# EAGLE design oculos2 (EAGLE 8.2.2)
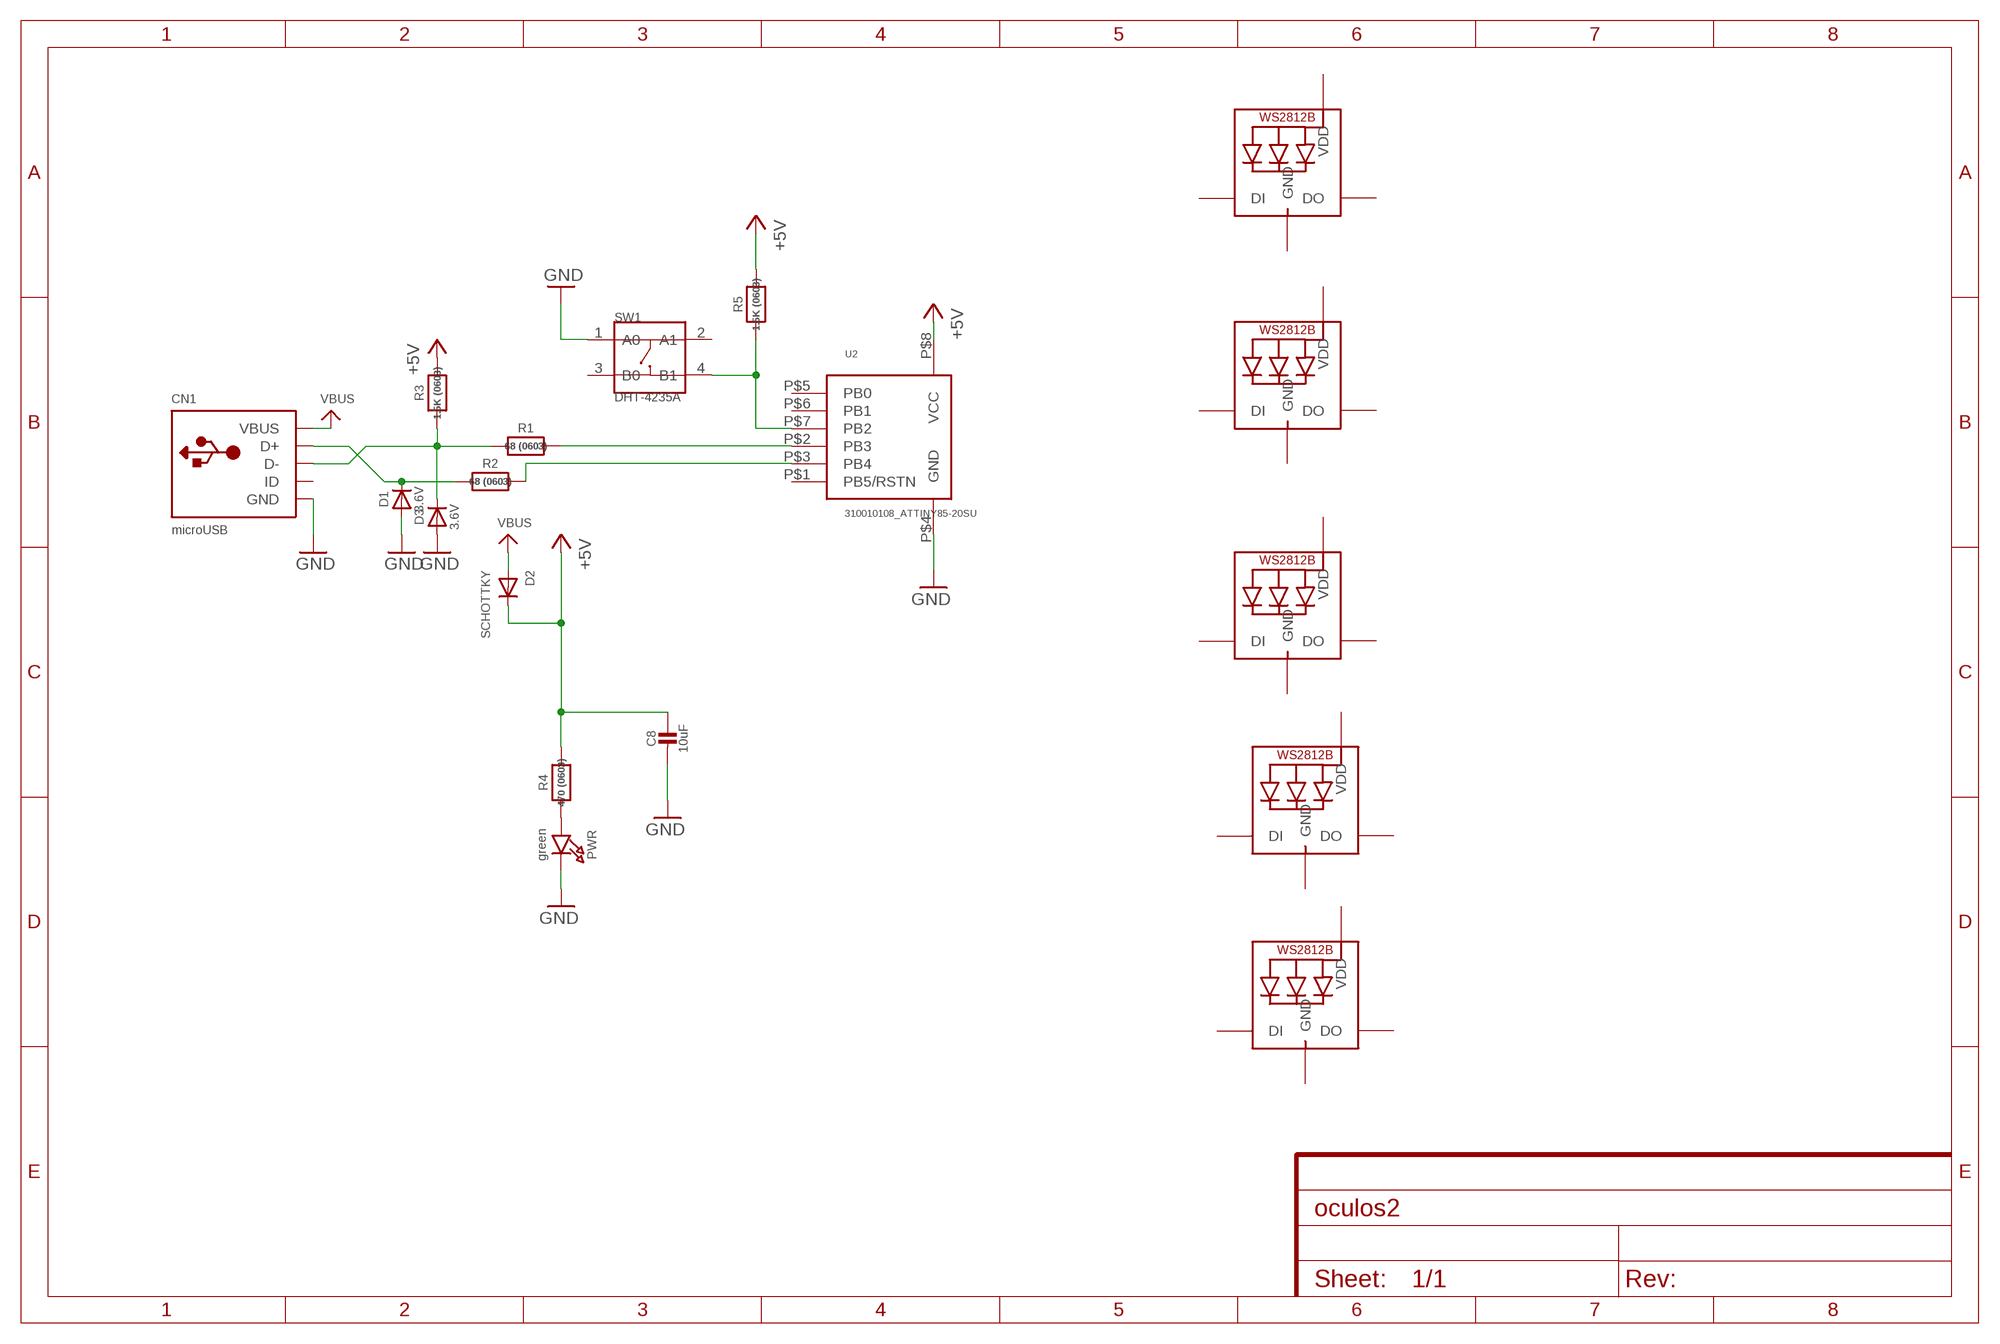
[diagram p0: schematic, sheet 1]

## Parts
C8  10uF  CAP_CERAMIC0805-NOOUTLINE  [0805-NO]
CN1  microUSB  USBMICRO_20329  [4UCONN_20329]
D1  3.6V  DIODESOD-323  [SOD-323]
D2  SCHOTTKY  DIODE_SOD-123FL  [SOD-123FL]
D3  3.6V  DIODESOD-323  [SOD-323]
LED1  WS2812B5050  [WS2812B]
LED2  WS2812B5050  [WS2812B]
LED3  WS2812B5050  [WS2812B]
LED4  WS2812B5050  [WS2812B]
LED5  WS2812B5050  [WS2812B]
PWR  green  LED0805_NOOUTLINE  [CHIPLED_0805_NOOUTLINE]
R1  68 (0603)  RESISTOR_0603_NOOUT  [0603-NO]
R2  68 (0603)  RESISTOR_0603_NOOUT  [0603-NO]
R3  1.5K (0603)  RESISTOR_0603_NOOUT  [0603-NO]
R4  470 (0603)  RESISTOR_0603_NOOUT  [0603-NO]
R5  1.5K (0603)  RESISTOR_0603_NOOUT  [0603-NO]
SW1  DHT-4235A  SMD-BUTTON-TOP-DHT-4235A(4P-4.2X3.2MM)  [SW4-SMD-4.2X3.2X2.5MM]
U2  310010108_ATTINY85-20SU  [SOIC8]

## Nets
+5V: C8.1 D2.C R3.2 R4.2 R5.2 U2.P$8(VCC)
B3: R1.2 U2.P$2(PB3)
GND: C8.2 CN1.BASE@1(GND) CN1.BASE@2(GND) CN1.GND CN1.SPRT@1(GND) CN1.SPRT@2(GND) CN1.SPRT@3(GND) CN1.SPRT@4(GND) D1.A D3.A PWR.C SW1.1(A0) U2.P$4(GND)
N$1: R5.1 SW1.4(B1) U2.P$7(PB2)
N$2: CN1.D+ D1.C R2.1
N$3: R2.2 U2.P$3(PB4)
N$5: CN1.D- D3.C R1.1 R3.1
N$6: PWR.A R4.1
VBUS: CN1.VBUS D2.A
Unconnected: CN1.ID LED1.2-DOUT(DO) LED1.4-DIN(DI) LED2.2-DOUT(DO) LED2.4-DIN(DI) LED3.2-DOUT(DO) LED3.4-DIN(DI) LED4.2-DOUT(DO) LED4.4-DIN(DI) LED5.2-DOUT(DO) LED5.4-DIN(DI) SW1.2(A1) SW1.3(B0) U2.P$1(PB5/RSTN) U2.P$5(PB0) U2.P$6(PB1)

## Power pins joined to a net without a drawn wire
GND: LED1.3-GND(GND) LED2.3-GND(GND) LED3.3-GND(GND) LED4.3-GND(GND) LED5.3-GND(GND)
VDD: LED1.1-VDD(VDD) LED2.1-VDD(VDD) LED3.1-VDD(VDD) LED4.1-VDD(VDD) LED5.1-VDD(VDD)

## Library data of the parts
C8 = microbuilder:CAP_CERAMIC: Ceramic Capacitors
CN1 = microbuilder:USB: USB Connectors USBMINIB - Surface Mount Female Mini-B USB Connector 4UConnector: 06564
D1 D3 = microbuilder:DIODE: Diode
D2 = adafruit:DIODE: Diode
LED1-LED5 = adafruit:WS2812B
PWR = microbuilder:LED: LED
R1-R5 = microbuilder:RESISTOR: Resistors
SW1 = Seeed-Switch-2016:SMD-BUTTON-TOP-DHT-4235A(4P-4.2X3.2MM): 311020045; MPN: DHT-4235A
U2 = Seeed-OPL-2017-01-IC-Akita:310010108_ATTINY85-20SU: Atmel;ATTINY85-20SU, SMD IC MCU;SOIC-8, SKU: 310010108

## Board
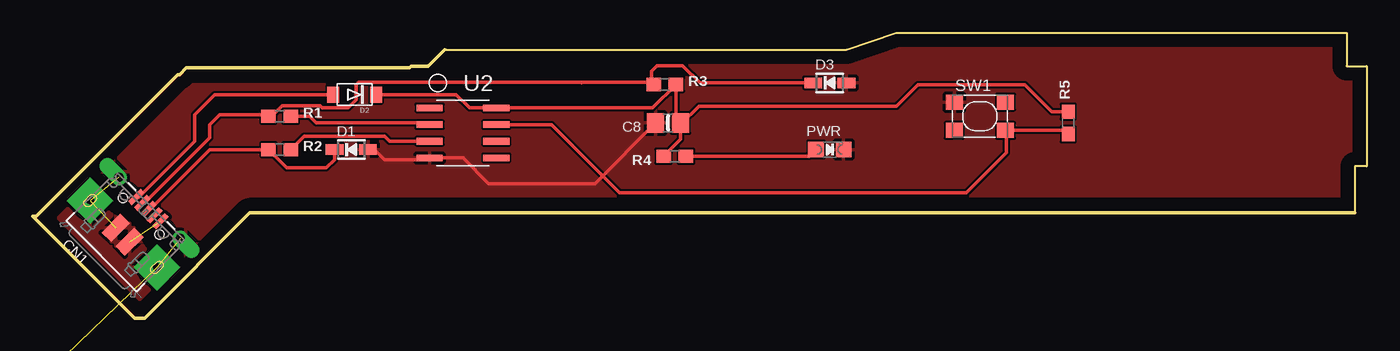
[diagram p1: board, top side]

Size 101.6 x 21.72 mm. Coordinates in mm from the lower left corner, seen from the top.
Outline: 31.5,20.45 61.98,20.45 65.79,21.72 100.08,21.72 100.08,19.18 101.6,19.18 101.6,11.56 100.71,11.56 100.71,8.13
Outline: 100.71,8 16.51,8 8.51,0 7.75,0 0,7.75 0.25,7.75 11.05,18.54 11.18,18.54 11.68,19.05 28.7,19.05 28.83,19.18 30.1,19.18 31.37,20.45
Copper layers (1*16): Top 0.035mm / dielectric 1.5mm / Bottom 0.035mm
Design rules "default": minimum track width 6mil, minimum drill 0.35mm, track to track 6mil, track to pad 6mil, pad to pad 6mil, via to via 6mil, smd to smd 6mil, copper to edge 40mil, drill to drill 6mil, minimum pad ring 10mil, minimum via ring 8mil, stop-mask expansion 4mil, vias tented up to drill 0mil, thermal gap 10mil

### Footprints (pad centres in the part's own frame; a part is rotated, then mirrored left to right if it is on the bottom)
0805-NO = smd 1.3 x 1.5: 1 -0.95,0; 2 0.95,0
4UCONN_20329 = smd 1 x 2: BASE@1 -0.75,-2; BASE@2 0.75,-2 | smd 0.4 x 1.35: D+ 0,0.775; D- -0.65,0.775; GND 1.3,0.775; ID 0.65,0.775; VBUS -1.3,0.775 | drill 0.7 offset: SPRT@1 -3.3,0.9; SPRT@2 3.3,0.9 | drill 0.6 pad 2.5 square: SPRT@3 -3.6,-1.9; SPRT@4 3.6,-1.9 | hole 0.7: -1.95,0; 1.95,0
SOD-323 = smd 1.35 x 0.8: A 1.27,0; C -1.27,0
SOD-123FL = smd 0.91 x 1.22: A 1.637,0; C -1.637,0
WS2812B = smd 1.5 x 0.9: 1-VDD 2.45,-1.65; 2-DOUT 2.45,1.65; 3-GND -2.45,1.65; 4-DIN -2.45,-1.65
CHIPLED_0805_NOOUTLINE = smd 1.2 x 1.2: A 0,-1.05; C 0,1.05
0603-NO = smd 1.1 x 1: 1 -0.85,0; 2 0.85,0
SW4-SMD-4.2X3.2X2.5MM = smd 1.3 x 1.15: 1 -1.95,1.075; 2 1.95,1.075; 3 -1.95,-1.075; 4 1.95,-1.075
SOIC8 = smd 2 x 0.5: P$1 -2.54,1.905; P$2 -2.54,0.635; P$3 -2.54,-0.635; P$4 -2.54,-1.905; P$5 2.54,-1.905; P$6 2.54,-0.635; P$7 2.54,0.635; P$8 2.54,1.905

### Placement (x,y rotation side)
C8  48.39,14.86 180 top
CN1  8.26,7.75 315 top
D1  24.26,12.83 0 top
D2  24.51,17.02 180 top
D3  60.71,17.91 0 top
LED1  not placed on the board
LED2  not placed on the board
LED3  not placed on the board
LED4  not placed on the board
LED5  not placed on the board
PWR  60.71,12.83 270 top
R1  18.8,15.37 0 top
R2  18.8,12.83 0 top
R3  48.13,17.78 0 top
R4  48.89,12.32 180 top
R5  78.87,14.86 90 top
SW1  72.14,15.37 0 top
U2  32.77,14.1 0 top

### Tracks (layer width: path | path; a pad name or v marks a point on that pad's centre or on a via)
+5V
  Top 0.254: D2.C 32.26,17.02 33.27,16 U2.P$8 47.2,16 R3.2 48.98,15.21 C8.1 49.34,14.74 | 49.34,14.74 49.34,13.61 R4.2 | R5.2 77.64,15.71 75.56,17.78 67.44,17.78 65.79,16.13 50.73,16.13 49.34,14.74
B3
  Top 0.254: R1.2 21.08,15.37 21.59,14.86 30.47,14.86 | 30.47,14.86 30.61,14.86 30.86,14.61 | U2.P$2 30.35,14.73 30.47,14.86
GND  (9 unrouted)
  Top 0.254: D1.A 26.04,12.83 26.8,12.07 30.1,12.07 U2.P$4 32.77,12.19 34.72,10.24 42.81,10.24 C8.2
  pour Top: 100.97,8.13 16.26,8.13 15.88,7.75 15.62,7.75 8.26,0.38 7.75,0.38 0.13,8 0.76,8 12.07,19.3 29.34,19.3 32.26,22.23 101.09,21.46
N$1
  Top 0.254: 74.17,14.37 SW1.4 78.58,14.29 R5.1 | U2.P$7 39.5,14.73 44.7,9.53 71.12,9.53 74.17,12.57 74.17,14.37 | 74.17,14.37 74.21,14.41
N$2
  Top 0.254: D1.C 22.99,12.07 22.35,11.43 19.34,11.43 R2.1 13.46,12.83 8.93,8.29 CN1.D+
N$3
  Top 0.254: U2.P$3 27.18,13.46 26.8,13.84 20.66,13.84 R2.2
N$5
  Top 0.254: 17.96,15.37 R1.1 | 17.96,15.37 18.2,15.37 18.98,16.15 21.88,16.15 22.02,16 24,16 24.64,16.64 24.64,17.78 24.82,17.96 41.73,17.96 | 41.73,17.96 41.78,17.91 | 41.73,17.96 47.1,17.96 R3.1 47.12,17.95 47.12,18.8 47.55,19.23 49.48,19.23 50.8,17.91 D3.C | CN1.D- 8.5,8.76 13.46,13.72 13.46,14.73 14.22,15.49 17.83,15.49 17.96,15.37
N$6
  Top 0.254: R4.1 59.15,12.32 PWR.A
VBUS
  Top 0.254: CN1.VBUS 8.07,9.21 12.32,13.46 12.32,15.49 13.84,17.02 D2.A
VDD  (4 unrouted)

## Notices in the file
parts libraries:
SparkFun-Aesthetics: Licensing: Creative Commons ShareAlike 4.0 International - https://creativecommons.org/licenses/by-sa/4.0
microbuilder: This work is placed in the public domain, and may be freely used for commercial and non-commercial work with the following conditions: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
